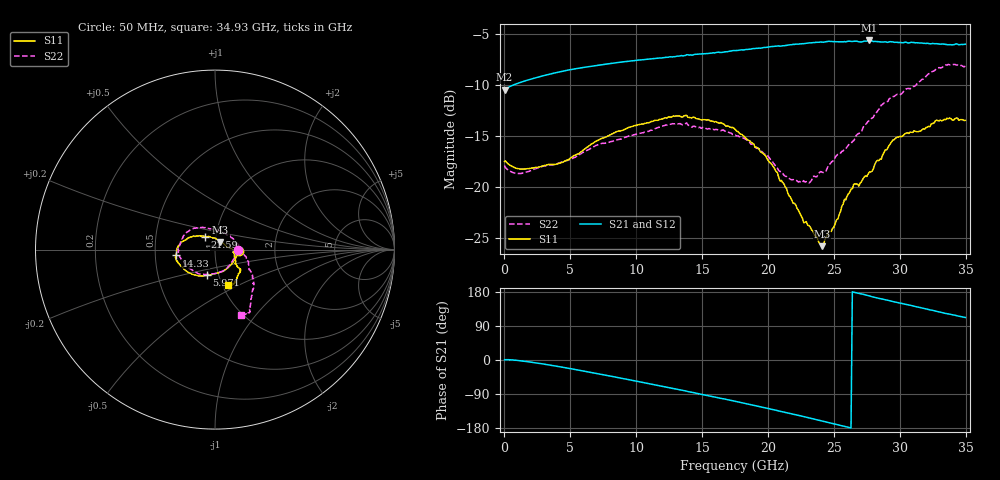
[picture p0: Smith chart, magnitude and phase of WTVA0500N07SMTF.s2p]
! 50 ohm 2-Port S-parameters measured by Modelithics Inc support@modelithics.com  Tampa, FL USA 813-866-6335 (February 2024)
! Smiths Interconnect,  5dB P/N: WTVA0500N07SMTF, Temperature: -50 C
! Board: 10 mil Rogers 4350B, Mounting Pad Dimensions: Length: 15 mils, Width: 25 mils, Gap: 40 mils.
# Hz S RI R 50
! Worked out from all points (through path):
!   352 points, 50 MHz to 34.93 GHz, reference 50 ohm
!   highest |S21| = -5.60 dB at 27.66 GHz (marker M1); lowest = -10.4 dB at 50 MHz (marker M2)
!   group delay of S21, straight-line fit = 20.6 ps
!   lowest |S11| = -25.8 dB at 24.08 GHz (marker M3), VSWR 1.11, Z = 52.9 + j4.41 ohm
!   |S11| at or under -10 dB: start of sweep to end of sweep
!   |S22| runs from -19.6 to -7.9 dB; largest |S21 - S12| = 0.0028
!   S11 on the Smith chart (normalised r, x): 50 MHz: 1.31, -0.01; 5.971 GHz: 0.87, -0.26; 14.33 GHz: 0.64, -0.04; 21.59 GHz: 0.89, +0.13; 34.93 GHz: 1.07, -0.44
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5e7  0.1332 -0.00525  0.3005 0.00266  0.3004 0.00248  0.1273 -0.00498
1.2945e9  0.1018 -0.0681  0.3272 -0.0126  0.3271 -0.0126  0.0931 -0.0702
4.18e9  0.0175 -0.1294  0.3503 -0.1108  0.3501 -0.1108  0.0111 -0.1308
5.8715e9  -0.0433 -0.1431  0.3396 -0.1821  0.3395 -0.1821  -0.0486 -0.1383
5.971e9  -0.0472 -0.1435  0.3384 -0.1864  0.3383 -0.1864  -0.0518 -0.1385
8.558e9  -0.1272 -0.1379  0.2846 -0.2928  0.2843 -0.2929  -0.1252 -0.1161
1.1742e10  -0.1982 -0.0825  0.163 -0.3981  0.1625 -0.3982  -0.1903 -0.0496
1.4329e10  -0.218 -0.0328  0.0324 -0.4448  0.032 -0.4447  -0.1982 0.0186
1.7513e10  -0.1872 0.0414  -0.154 -0.442  -0.1541 -0.4419  -0.1474 0.1032
1.98015e10  -0.121 0.0749  -0.2884 -0.3895  -0.2878 -0.3898  -0.0774 0.1234
2.15925e10  -0.0552 0.0715  -0.3847 -0.3179  -0.3845 -0.3179  0.0034 0.1101
2.2687e10  -0.0144 0.0652  -0.4352 -0.2585  -0.4351 -0.2583  0.0532 0.0935
2.3085e10  -0.00418 0.0646  -0.4533 -0.2349  -0.4531 -0.235  0.066 0.0811
2.33835e10  0.00555 0.0609  -0.4645 -0.2161  -0.4644 -0.216  0.078 0.0814
2.408e10  0.03 0.0416  -0.4874 -0.1668  -0.4873 -0.1668  0.1061 0.0522
2.6468e10  0.1031 -0.00234  -0.5198 0.00944  -0.5196 0.00873  0.1653 -0.0343
2.6866e10  0.0999 -0.0145  -0.5152 0.0413  -0.515 0.0414  0.1751 -0.0544
2.7662e10  0.1106 -0.0427  -0.5154 0.0992  -0.5151 0.0997  0.1884 -0.0974
2.91545e10  0.1261 -0.0987  -0.4751 0.2038  -0.4748 0.204  0.215 -0.1651
2.97515e10  0.139 -0.1077  -0.4533 0.2425  -0.453 0.2426  0.2142 -0.1885
3.2836e10  0.115 -0.1783  -0.3072 0.4013  -0.3084 0.4002  0.1977 -0.3299
3.49255e10  0.075 -0.1989  -0.1897 0.4656  -0.188 0.4661  0.1454 -0.3645
